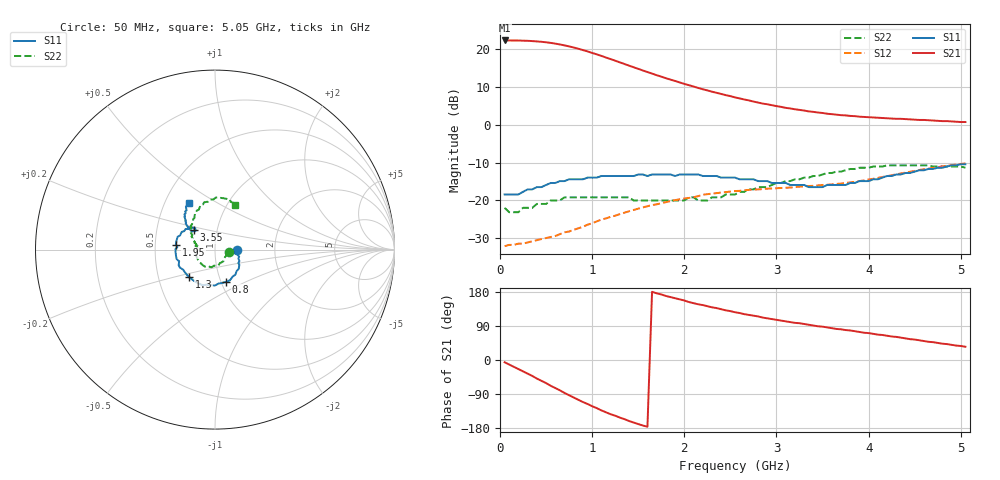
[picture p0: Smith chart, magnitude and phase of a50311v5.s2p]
!  INA-50311 S PARAMETERS
!  Vd = 5 V  LAST UPDATED 12-19-94
# ghz s ma r 50
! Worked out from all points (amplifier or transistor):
!   101 points, 50 MHz to 5.05 GHz, reference 50 ohm
!   highest |S21| = 22.2 dB at 50 MHz (marker M1)
!   |S21| within 3 dB of that: start of sweep to 964.5 MHz
!   unconditionally stable (mu >= 1): start of sweep to end of sweep
!   at 850 MHz: K = 1.34, MAG = 20.1 dB, |S12| = -27.3 dB
!   at 2.55 GHz: K = 1.73, MAG = 7.4 dB, |S12| = -17.5 dB
!   at 5.05 GHz: K = 1.47, MAG = 1.4 dB, |S12| = -10.2 dB
!   S11 on the Smith chart (normalised r, x): 50 MHz: 1.27, -0.01; 800 MHz: 1.06, -0.39; 1.3 GHz: 0.72, -0.23; 1.95 GHz: 0.64, +0.04; 3.55 GHz: 0.77, +0.17; 5.05 GHz: 0.66, +0.38
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0.05  0.12 -2.0  12.82 -6.0  0.025 5.0  0.08 -11.0
0.15  0.12 -8.0  12.8 -18.0  0.026 13.0  0.07 -35.0
0.25  0.13 -13.0  12.73 -30.0  0.027 20.0  0.08 -54.0
0.35  0.14 -21.0  12.58 -42.0  0.029 27.0  0.08 -70.0
0.45  0.15 -30.0  12.31 -55.0  0.031 33.0  0.09 -86.0
0.55  0.17 -39.0  11.91 -68.0  0.033 39.0  0.1 -101.0
0.6  0.17 -45.0  11.65 -74.0  0.034 42.0  0.1 -107.0
0.7  0.18 -57.0  11.04 -87.0  0.038 47.0  0.11 -120.0
0.8  0.19 -71.0  10.35 -99.0  0.041 51.0  0.11 -131.0
0.9  0.19 -84.0  9.57 -111.0  0.045 54.0  0.11 -141.0
1  0.2 -98.0  8.78 -122.0  0.05 56.0  0.11 -149.0
1.1  0.21 -109.0  8.02 -133.0  0.056 58.0  0.11 -156.0
1.3  0.21 -133.0  6.6 -152.0  0.066 60.0  0.11 -168.0
1.55  0.22 -157.0  5.16 -173.0  0.081 60.0  0.1 -177.0
1.75  0.22 -174.0  4.28 173.0  0.092 58.0  0.1 177.0
1.95  0.22 173.0  3.59 160.0  0.104 56.0  0.1 172.0
2.15  0.22 161.0  3.04 147.0  0.114 55.0  0.1 163.0
2.55  0.2 145.0  2.28 126.0  0.133 48.0  0.12 159.0
3.4  0.15 136.0  1.47 91.0  0.156 43.0  0.21 125.0
3.55  0.16 138.0  1.39 86.0  0.161 43.0  0.23 119.0
4.25  0.21 139.0  1.2 62.0  0.215 45.0  0.29 87.0
5.05  0.3 119.0  1.08 35.0  0.308 31.0  0.27 66.0
